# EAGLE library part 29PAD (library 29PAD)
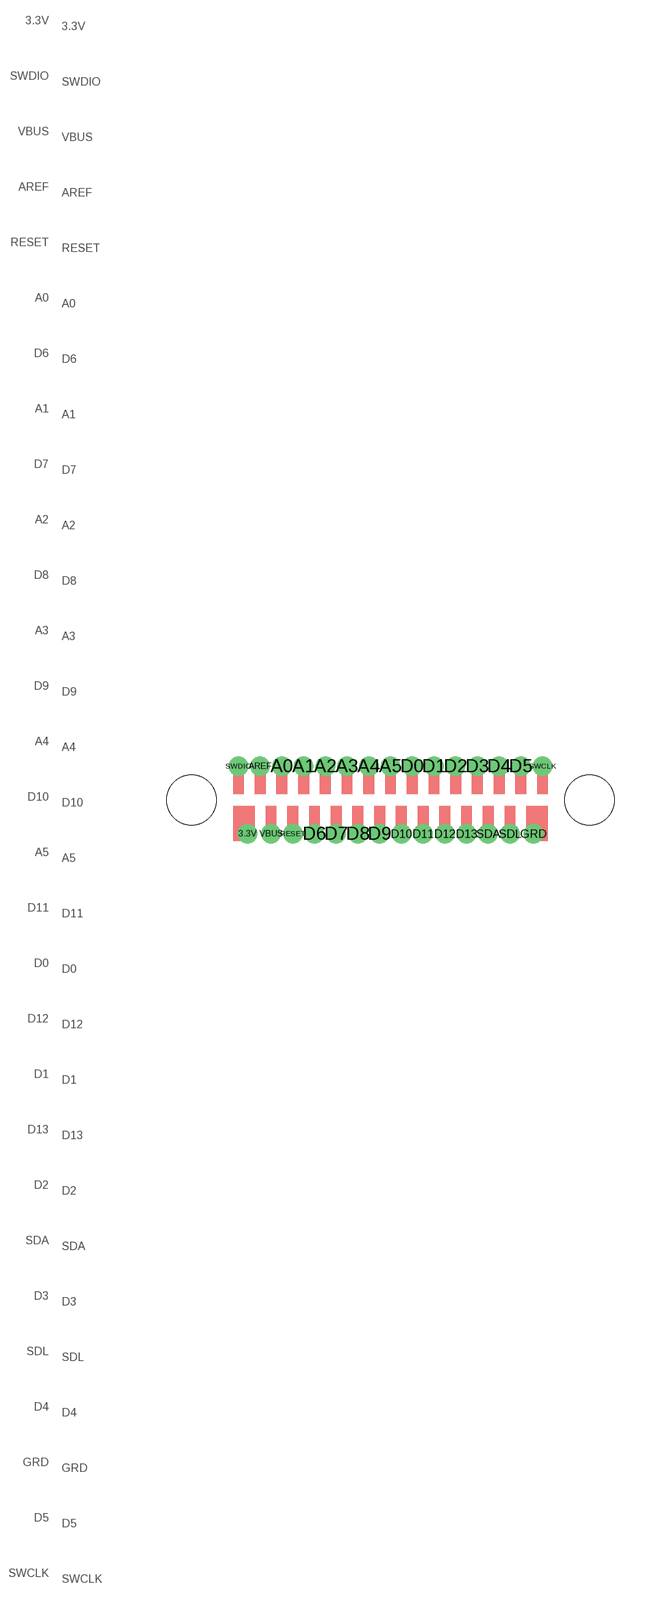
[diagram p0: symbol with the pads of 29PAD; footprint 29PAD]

Designator prefix -

## 29PAD  [29PAD]
3.3V  3.3V
A0  A0
A1  A1
A2  A2
A3  A3
A4  A4
A5  A5
AREF  AREF
D0  D0
D1  D1
D2  D2
D3  D3
D4  D4
D5  D5
D6  D6
D7  D7
D8  D8
D9  D9
D10  D10
D11  D11
D12  D12
D13  D13
GRD  GRD
RESET  RESET
SDA  SDA
SDL  SDL
SWCLK  SWCLK
SWDIO  SWDIO
VBUS  VBUS

## Footprint 29PAD (pad centres in mm)
drill 0.3 pad 0.3: 3.3V -5.925,-1.4; A0 -4.5,1.4; A1 -3.6,1.4; A2 -2.7,1.4; A3 -1.8,1.4; A4 -0.9,1.4; A5 0,1.4; AREF -5.4,1.4; D0 0.9,1.4; D1 1.8,1.4; D2 2.7,1.4; D3 3.6,1.4; D4 4.5,1.4; D5 5.4,1.4; D6 -3.15,-1.4; D7 -2.25,-1.4; D8 -1.35,-1.4; D9 -0.45,-1.4; D10 0.45,-1.4; D11 1.35,-1.4; D12 2.25,-1.4; D13 3.15,-1.4; GRD 5.925,-1.4; RESET -4.05,-1.4; SDA 4.05,-1.4; SDL 4.95,-1.4; SWCLK 6.3,1.4; SWDIO -6.3,1.4; VBUS -4.95,-1.4
hole 2.05 at -8.25,0
hole 2.05 at 8.25,0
